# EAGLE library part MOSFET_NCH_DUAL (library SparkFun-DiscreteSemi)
Dual N-Channel 30-VDS MOSFET Link to datasheet SparkFun Products: SparkFun Mini FET Shield
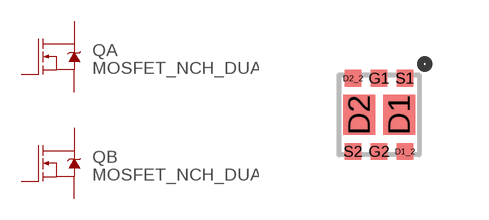
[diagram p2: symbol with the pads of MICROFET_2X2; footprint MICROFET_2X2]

Designator prefix Q; gates A=LABELED-NMOS B=LABELED-NMOS

## MOSFET_NCH_DUAL-FDMA1024NZ (PROD_ID: TRANS-09516; VALUE: 5A/20V/54mΩ)  [MICROFET_2X2]
D1  A:D
D1_2  A:D
D2  B:D
D2_2  B:D
G1  A:G
G2  B:G
S1  A:S
S2  B:S

## Footprint MICROFET_2X2 (pad centres in mm)
1206-8 ChipFET Source: http://www.vishay.com/docs/72593/72593.pdf http://www.vishay.com/docs/71151/71151.pdf
smd 0.8 x 1: D1 0.5,0; D2 -0.5,0
smd 0.42 x 0.42: D1_2 0.65,-0.915; D2_2 -0.65,0.915; G1 0,0.915; G2 0,-0.915; S1 0.65,0.915; S2 -0.65,-0.915

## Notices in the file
Licensing: Creative Commons ShareAlike 4.0 International - https://creativecommons.org/licenses/by-sa/4.0
